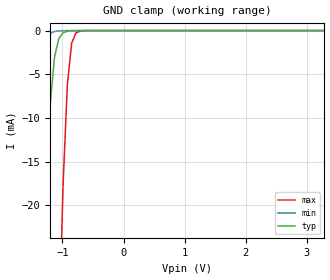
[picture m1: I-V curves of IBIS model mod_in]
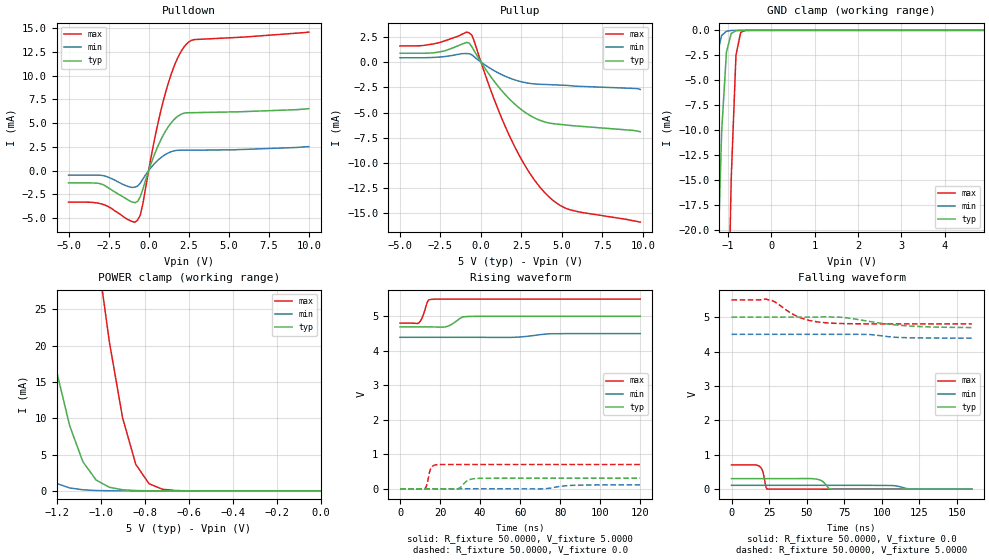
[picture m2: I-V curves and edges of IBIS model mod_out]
| IBIS (I/O, Buffer, Information, Specification) Model, officially
| electronic behavioral standard for Buffer structures of digital pins.
[IBIS ver]  4.0
[File name] hcc40109b_3v3_rev1.ibs
[File Rev]  1.0
[Date]   22 Oct 2020
[Source]   CAD & Design Services (Catania) - STMicroelectronics
[Notes]
   (Note1) This IBIS model is the model of the product with package
   (Flat16 package elements);
   (Note3) This IBIS model is extracted with nominal Vdd1=3.3V and Vdd2=5.0V;
   (Note2)  This IBIS model has some Notes about the non-monotonicity
   of the I-V curves, but they are not indicative of problems
   inside the model;
[Copyright] (c) 2020 STMicroelectronics
|   Component HCC40109B
[Component] HCC40109B
[Manufacturer] STMicroelectronics
[Package]
| variable   typ   min   max
R_pkg   0.0   0.0   0.0
L_pkg   0.0H   0.0H   0.0H
C_pkg   0.0F   0.0F   0.0F
[Pin]   signal_name   model_name   R_pin   L_pin   C_pin
1   VCC   POWER   78.8m   2.61nH   1.01pF
2   EN_A   mod_in   54.2m   1.20nH   1.08pF
3   A   mod_in   26.6m   0.75nH   1.04pF
4   E   mod_out   26.6m   0.75nH   1.04pF
5   F   mod_out   26.6m   0.75nH   1.04pF
6   B   mod_in   26.6m   0.75nH   1.04pF
7   EN_B   mod_in   54.2m   1.20nH   1.08pF
8   VSS   GND   78.8m   2.61nH   1.01pF
9   EN_C   mod_in   78.8m   2.61nH   1.01pF
10   C   mod_in   54.2m   1.20nH   1.08pF
11   G   mod_out   26.6m   0.75nH   1.04pF
12   NC   NC   26.6m   0.75nH   1.04pF
13   H   mod_out   26.6m   0.75nH   1.04pF
14   D   mod_in   26.6m   0.75nH   1.04pF
15   EN_D   mod_in   54.2m   1.20nH   1.08pF
16   VDD   POWER   78.8m   2.61nH   1.01pF
| Models and submodels in the file (2): mod_in (Input), mod_out (3-state)
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|   Model mod_in
[Model]   mod_in
Model_type Input
Vinl   =   1.000V
Vinh   =   2.300V
C_comp   0.640pF   0.611pF   0.702pF
[Temperature Range]  25.0000   85.0000   -40.0000
[Voltage Range]   3.3000V   3.0000V   3.6000V
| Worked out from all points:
|   GND clamp passes 1 mA (typ) near -1.06 V on its own axis
[GND_clamp]
|Voltage   I(typ)   I(min)   I(max)
-3.3V     -600.2mA   -423.5mA   -912.9mA
-1.62V    -100.3mA   -32.45mA   -236.3mA
-1.55V    -81.57mA   -21.22mA   -209.2mA
-1.41V    -46.58mA   -5.827mA   -155.9mA
-1.34V    -31.09mA   -2.355mA   -129.8mA
-1.27V    -17.96mA   -849.1uA   -104.3mA
-1.2V     -8.363mA   -293.2uA   -79.69mA
-1.06V    -903.8uA   -34.24uA   -35.14mA
-990mV    -253.7uA   -11.04uA   -17.61mA
-920mV    -69.67uA   -3.509uA   -6.157mA
-780mV    -4.46uA    -348.2nA   -281.2uA
3.28V     1pA        1pA        1pA
|   Model mod_out
[Model]   mod_out
Model_type 3-state
Polarity   Non-Inverting
|Vinl   =   1.500V
|Vinh   =   3.500V
Vmeas  =   2.500V
Cref   =   50.0pF
Rref   =   200k
Vref   =   5.0
C_comp   1.466pF   1.400pF   1.607pF
[Temperature Range]  25.0000   85.0000   -40.0000
[Voltage Range]   5.0000V   4.5000V   5.5000V
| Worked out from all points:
|   slope of the pulldown table from 0 to 0.75 V, typ, clamps not added: 235 ohm
|   slope of the pullup table from 0 to 0.75 V, typ, clamps not added: 426 ohm
|   GND clamp passes 1 mA (typ) near -0.97 V on its own axis
|   POWER clamp passes 1 mA (typ) near -0.99 V on its own axis
|   rising waveform, R_fixture 50.0000, V_fixture 5.0000: 20-80 % time 4.6ns typ, 9.36ns min, 2.43ns max; typ from 4.69 V to 5 V
|   rising waveform, R_fixture 50.0000, V_fixture 0.0: 20-80 % time 3.41ns typ, 7.94ns min, 1.73ns max; typ from 0 V to 0.307 V
|   falling waveform, R_fixture 50.0000, V_fixture 0.0: 20-80 % time 4.09ns typ, 5.79ns min, 2.16ns max; typ from 0.307 V to 0 V
|   falling waveform, R_fixture 50.0000, V_fixture 5.0000: 20-80 % time 30.6ns typ, 13.8ns min, 17ns max; typ from 5 V to 4.7 V
[Pulldown]
|Voltage   I(typ)   I(min)   I(max)
-5V       -1.296mA   -472uA     -3.32mA
-2.92V    -1.425mA   -505uA     -3.521mA
-1.16V    -3.212mA   -1.733mA   -5.257mA
-680mV    -3.221mA   -1.617mA   -5.189mA
-520mV    -2.736mA   -1.314mA   -4.687mA
-360mV    -1.966mA   -895.5uA   -3.502mA
440mV     2.015mA    865.7uA    3.865mA
1.08V     4.226mA    1.728mA    8.355mA
1.4V      5.01mA     1.983mA    10.1mA
1.88V     5.787mA    2.146mA    12.08mA
2.52V     6.089mA    2.153mA    13.55mA
10V       6.521mA    2.522mA    14.58mA
[Pullup]
|Voltage   I(typ)   I(min)   I(max)
-5V       874uA      428uA      1.602mA
-2.8V     945.2uA    475uA      1.847mA
-880mV    1.951mA    844.2uA    2.972mA
-720mV    1.867mA    822.2uA    2.889mA
-560mV    1.513mA    714.7uA    2.659mA
720mV     -1.696mA   -761.5uA   -3.287mA
1.84V     -3.79mA    -1.625mA   -7.579mA
2.8V      -5.057mA   -2.055mA   -10.46mA
3.92V     -5.921mA   -2.215mA   -12.9mA
4.72V     -6.145mA   -2.268mA   -14.02mA
5.52V     -6.28mA    -2.343mA   -14.64mA
9.84V     -6.904mA   -2.711mA   -15.86mA
[GND_clamp]
|Voltage   I(typ)   I(min)   I(max)
-5V       -967.4mA   -756.6mA   -1.31A
-1.48V    -70.88mA   -21.63mA   -165.8mA
-1.37V    -47.28mA   -9.104mA   -132.2mA
-1.26V    -26.21mA   -2.519mA   -99.36mA
-1.15V    -10.13mA   -513.4uA   -67.85mA
-1.04V    -2.193mA   -93.39uA   -38.74mA
-930mV    -314.2uA   -15.65uA   -14.94mA
-820mV    -37.45uA   -2.58uA    -2.495mA
-710mV    -4.289uA   -422.7nA   -192.5uA
-600mV    -490.3nA   -69.34nA   -12.44uA
-490mV    -56.46nA   -11.45nA   -796.9nA
4.9V      10.17pA    2.62nA     8.6pA
[POWER_clamp]
|Voltage   I(typ)   I(min)   I(max)
-4.98V    962.2mA    752.2mA    1.304A
-1.56V    88.93mA    33.39mA    190.5mA
-1.5V     75.3mA     24.36mA    171.9mA
-1.32V    37.22mA    5.284mA    117.1mA
-1.26V    26.14mA    2.452mA    99.33mA
-1.14V    8.95mA     407.7uA    65.03mA
-1.02V    1.496mA    59.84uA    33.81mA
-960mV    501.1uA    22.7uA     20.52mA
-900mV    159.9uA    8.595uA    10.06mA
-840mV    50.14uA    3.253uA    3.652mA
-780mV    15.64uA    1.231uA    999.3uA
0V        14pA       13pA       15pA
[Ramp]
| variable   typ   min   max
dV/dt_r   0.1846/3.8441n   0.3045m/4.4738n   0.4251/2.1486n
dV/dt_f   0.1560/3.0221n   0.3004m/4.2230n   0.3973/16.2201n
R_load = 50.0000
[Rising Waveform]
R_fixture= 50.0000
V_fixture= 5.0000
V_fixture_min= 4.5000
V_fixture_max= 5.5000
|time   V(typ)   V(min)   V(max)
0s        4.692V     4.391V     4.802V
9.38ns    4.692V     4.391V     4.81V
11.06ns   4.692V     4.391V     4.96V
14.14ns   4.692V     4.391V     5.467V
15.54ns   4.692V     4.391V     5.49V
23.38ns   4.705V     4.391V     5.5V
32.9ns    4.991V     4.391V     5.5V
57.54ns   5V         4.393V     5.5V
75.18ns   5V         4.494V     5.5V
120ns     5V         4.5V       5.5V
[Rising Waveform]
R_fixture= 50.0000
V_fixture= 0.0
V_fixture_min= 0.0
V_fixture_max= 0.0
|time   V(typ)   V(min)   V(max)
0s        559.1pV    -7.784nV   508.4pV
12.18ns   -4.56uV    -212.7nV   -5.925mV
13.3ns    -1.02uV    -259.1nV   104mV
14.7ns    17.61uV    -305.3nV   475.7mV
15.54ns   54.31uV    -328.2nV   603.7mV
18.48ns   112.2uV    -385.6nV   699mV
28.7ns    -1.701mV   -503nV     704.9mV
33.74ns   239.1mV    6.721uV    705mV
37.94ns   298.7mV    22.29uV    705.1mV
119.8ns   307mV      112.2mV    705.2mV
[Falling Waveform]
R_fixture= 50.0000
V_fixture= 0.0
V_fixture_min= 0.0
V_fixture_max= 0.0
|time   V(typ)   V(min)   V(max)
0s        307mV      112.3mV    705.2mV
18.36ns   307mV      112.3mV    671.6mV
20.6ns    307mV      112.3mV    543mV
22.84ns   307mV      112.3mV    79.99mV
23.96ns   307mV      112.3mV    3.791mV
56.58ns   291.7mV    112.3mV    277.8uV
60.5ns    231.2mV    112.3mV    196.3uV
64.98ns   20.33mV    112.3mV    131.1uV
66.8ns    1.826mV    112.3mV    111.1uV
160ns     32.36uV    1.252uV    19.87nV
[Falling Waveform]
R_fixture= 50.0000
V_fixture= 5.0000
V_fixture_min= 4.5000
V_fixture_max= 5.5000
|time   V(typ)   V(min)   V(max)
0s        5V         4.5V       5.5V
22.7ns    5V         4.5V       5.525V
25.78ns   5V         4.5V       5.499V
43.7ns    5V         4.5V       5.023V
51.82ns   5V         4.5V       4.904V
60.22ns   5.006V     4.5V       4.846V
75.9ns    4.984V     4.5V       4.811V
92.7ns    4.869V     4.492V     4.804V
114.5ns   4.755V     4.405V     4.802V
160ns     4.697V     4.391V     4.802V
